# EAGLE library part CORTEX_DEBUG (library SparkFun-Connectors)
Cortex Debug Connector - 10 pin Supports JTAG debug, Serial Wire debug, and Serial Wire Viewer. PTH and SMD connector options available. General Connector Information Products: PTH Connector -via Digi-Key SparkFun PSoc SparkFun T
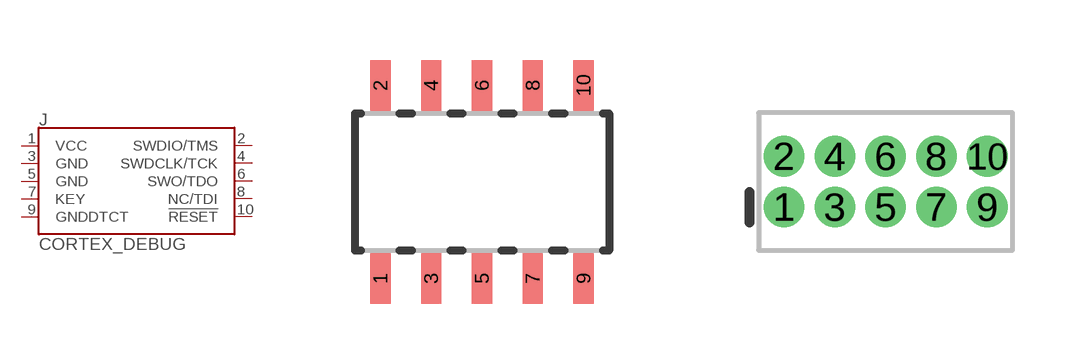
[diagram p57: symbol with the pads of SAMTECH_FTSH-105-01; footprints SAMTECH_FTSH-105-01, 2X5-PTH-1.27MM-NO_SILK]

Designator prefix J

## CORTEX_DEBUG_SMD  [SAMTECH_FTSH-105-01]
1  VCC
2  SWDIO/TMS
3  GND
4  SWDCLK/TCK
5  GND
6  SWO/TDO
7  KEY
8  NC/TDI
9  GNDDTCT
10  !RESET

## CORTEX_DEBUG_PTH_NS  [2X5-PTH-1.27MM-NO_SILK]
Pads as for SAMTECH_FTSH-105-01

## CORTEX_DEBUG_PTH  [2X5-PTH-1.27MM]
Pads as for SAMTECH_FTSH-105-01

## Footprint SAMTECH_FTSH-105-01 (pad centres in mm)
ARM Cortex Debug Connector (10-pin) Specifications: Pin count:10 Pin pitch:0.05" Datasheet referenced for footprint Example device(s): CORTEX_DEBUG
smd 0.508 x 1.27: 1 -2.54,-2.413; 2 -2.54,2.413; 3 -1.27,-2.413; 4 -1.27,2.413; 5 0,-2.413; 6 0,2.413; 7 1.27,-2.413; 8 1.27,2.413; 9 2.54,-2.413; 10 2.54,2.413

## Footprint 2X5-PTH-1.27MM-NO_SILK (pad centres in mm)
Plated Through Hole - 2x5 ARM Cortex Debug Connector (10-pin) tDoc (51) layer border represents maximum dimensions of plastic housing. Specifications: Pin count:10 Pin pitch:1.27mm Datasheet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
drill 0.508 pad 1: 1 -2.54,-0.635; 2 -2.54,0.635; 3 -1.27,-0.635; 4 -1.27,0.635; 5 0,-0.635; 6 0,0.635; 7 1.27,-0.635; 8 1.27,0.635; 9 2.54,-0.635; 10 2.54,0.635

## Footprint 2X5-PTH-1.27MM (pad centres in mm)
Plated Through Hole - 2x5 ARM Cortex Debug Connector (10-pin) tDoc (51) layer border represents maximum dimensions of plastic housing. Specifications: Pin count:10 Pin pitch:1.27mm Datasheet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
drill 0.508 pad 1: 1 -2.54,-0.635; 2 -2.54,0.635; 3 -1.27,-0.635; 4 -1.27,0.635; 5 0,-0.635; 6 0,0.635; 7 1.27,-0.635; 8 1.27,0.635; 9 2.54,-0.635; 10 2.54,0.635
